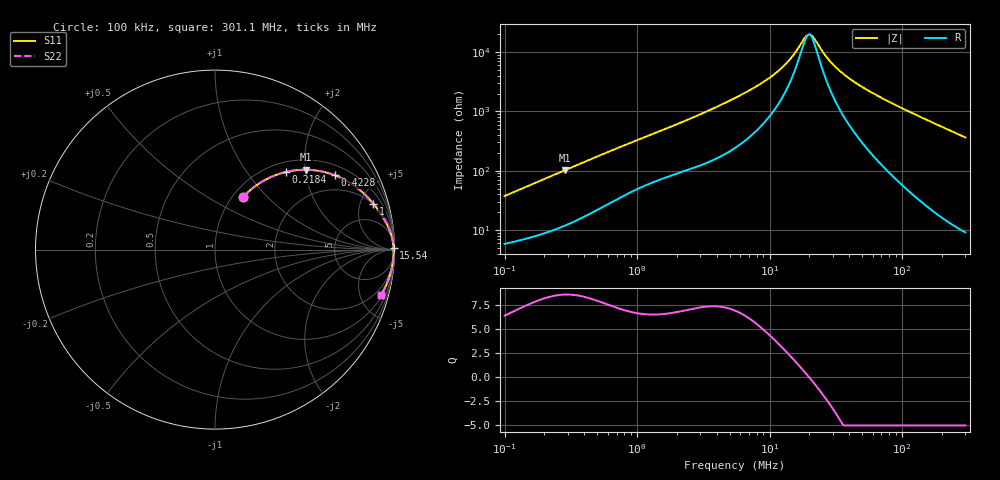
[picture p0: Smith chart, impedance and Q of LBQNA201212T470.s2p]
! LBQNA201212T470  S-PARAMETER MODEL  ( General Type )
! Model Generated by TAIYO YUDEN Corporation (http://www.ty-top.com)
! Version 1.0
! TAIYO YUDEN Control No. 191025NI43SB-FBB
! Copyright(c) 2019 TAIYO YUDEN CO.,LTD. All Rights Reserved.
! Product Description (link to TY-COMPAS)
! https://ds.yuden.co.jp/TYCOMPAS/or/detail?pn=LBQNA201212T470K&u=M
! Products Name : Inductors
! Characteristics :
!  Inductance : 47 uH , SRF(min) : 11 MHz , DC Resistance(max) : 4.81 Ohm
!  Rated Current : Saturation :90 mA , Temp Rise : 140 mA (20 degC)
!  Case Size : 2.0 x 1.25 / 0.079 x 0.049 [mm/inch] , Thickness : 1.25 / 0.049 [mm/inch]
!  (Conditions: Temperature = 25 degC , DC Bias Current/Voltage = 0A / 0V)
! External Node Assignments :
!  1  o---GGG---o  2
! GND o---------o GND
! Frequency Range : 0.1MHz  -  301.082333MHz  [ 402 STEP ]
# MHz S RI R 50
! Freq[MHz].  S11 Real  S11 Imag  S21 Real  S21 Imag  S12 Real  S12 Imag  S22 Real  S22 Imag
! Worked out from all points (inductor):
!   401 points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, 100 kHz to 301.1 MHz, reference 50 ohm
!   read as one part in series: L = 58.4 uH near 104.1 kHz
!   highest Q = 8.55 at 283.3 kHz (marker M1), where L = 56.6 uH
!   self-resonance near 19.77 MHz
!   S11 on the Smith chart (normalised r, x): 100 kHz: 1.12, +0.74; 218.4 kHz: 1.19, +1.57; 422.8 kHz: 1.36, +2.95; 1 MHz: 1.98, +6.48; 15.54 MHz: open; 301.1 MHz: 1.18, -7.27
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0.1  0.1584 0.2949  0.8416 -0.2949  0.8416 -0.2949  0.1584 0.2949
0.146298  0.2524 0.3724  0.7476 -0.3724  0.7476 -0.3724  0.2524 0.3724
0.218359  0.3963 0.4327  0.6037 -0.4327  0.6037 -0.4327  0.3963 0.4327
0.283289  0.5063 0.4449  0.4937 -0.4449  0.4937 -0.4449  0.5063 0.4449
0.382543  0.6313 0.4265  0.3687 -0.4265  0.3687 -0.4265  0.6313 0.4265
0.422828  0.6694 0.4136  0.3306 -0.4136  0.3306 -0.4136  0.6694 0.4136
0.643864  0.7986 0.3389  0.2014 -0.3389  0.2014 -0.3389  0.7986 0.3389
1.000281  0.8828 0.2549  0.1172 -0.2549  0.1172 -0.2549  0.8828 0.2549
1.463388  0.9277 0.1933  0.0723 -0.1933  0.0723 -0.1933  0.9277 0.1933
5.487097  0.9882 0.0575  0.0118 -0.0575  0.0118 -0.0575  0.9882 0.0575
10.41448  0.9935 0.0243  0.00651 -0.0243  0.00651 -0.0243  0.9935 0.0243
12.9808  0.9942 0.0155  0.00576 -0.0155  0.00576 -0.0155  0.9942 0.0155
15.54432  0.9947 0.00878  0.00534 -0.00878  0.00534 -0.00878  0.9947 0.00878
18.99061  0.995 0.00162  0.00504 -0.00162  0.00504 -0.00162  0.995 0.00162
19.76661  0.995 0.000206  0.005 -0.000206  0.005 -0.000206  0.995 0.000206
20.99048  0.9951 -0.00193  0.00495 0.00193  0.00495 0.00193  0.9951 -0.00193
27.23201  0.9951 -0.0114  0.00485 0.0114  0.00485 0.0114  0.9951 -0.0114
34.62902  0.995 -0.0209  0.005 0.0209  0.005 0.0209  0.995 -0.0209
48.67258  0.9942 -0.0366  0.00575 0.0366  0.00575 0.0366  0.9942 -0.0366
80.29753  0.991 -0.068  0.00903 0.068  0.00903 0.068  0.991 -0.068
158.6319  0.9754 -0.1389  0.0246 0.1389  0.0246 0.1389  0.9754 -0.1389
301.0823  0.9243 -0.2523  0.0757 0.2523  0.0757 0.2523  0.9243 -0.2523
